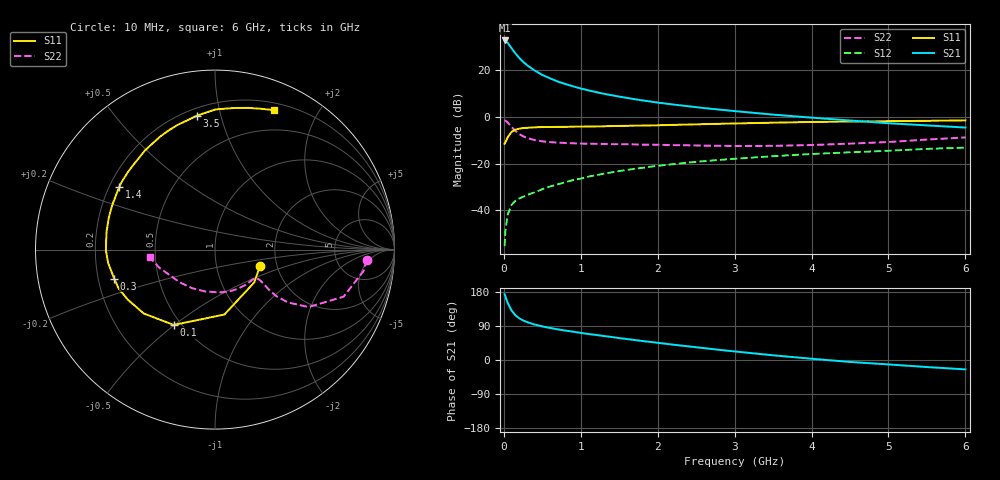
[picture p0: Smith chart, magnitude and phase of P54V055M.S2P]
! SIEMENS Small Signal Semiconductors
! BFP183
! Si NPN RF Bipolar Junction Transistor in SOT143
! VCE = 4 V  IC = 55 mA
! Common Emitter S-Parameters:  March  1996
# GHz  S  MA  R  50
!  f  S11  S21  S12  S22
! GHz  MAG  ANG  MAG  ANG  MAG  ANG  MAG  ANG
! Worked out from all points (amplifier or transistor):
!   36 points, 10 MHz to 6 GHz, reference 50 ohm
!   highest |S21| = 32.8 dB at 10 MHz (marker M1)
!   |S21| within 3 dB of that: start of sweep to 93.16 MHz
!   unconditionally stable (mu >= 1): start of sweep to 17.92 MHz; 311.2 MHz to end of sweep
!   at 250 MHz: K = 0.89, MSG = 28.9 dB, |S12| = -34.2 dB
!   at 1.4 GHz: K = 1.39, MAG = 12.8 dB, |S12| = -23.8 dB
!   at 6 GHz: K = 1.07, MAG = 2.7 dB, |S12| = -13.2 dB
!   S11 on the Smith chart (normalised r, x): 10 MHz: 1.63, -0.33; 100 MHz: 0.46, -0.50; 300 MHz: 0.27, -0.13; 1.4 GHz: 0.24, +0.28; 3.5 GHz: 0.25, +0.85; 6 GHz: 0.27, +1.47
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0.01  0.2669 -20.4  43.59 173.6  0.0017 72.9  0.8469 -3.8
0.02  0.285 -39.9  43.19 167.7  0.0036 72.5  0.8354 -8.3
0.05  0.3655 -81.7  38.92 150.5  0.0081 70.2  0.763 -20.1
0.1  0.4785 -118.7  29.74 130.7  0.013 54.0  0.6111 -31.6
0.15  0.5332 -138.1  23.05 118.2  0.016 51.0  0.5015 -35.9
0.2  0.5604 -150.2  18.42 110.1  0.0179 49.1  0.4302 -37.2
0.25  0.5786 -157.9  15.23 104.4  0.0194 51.7  0.385 -36.9
0.3  0.5844 -163.9  12.93 100.2  0.0211 53.2  0.3555 -36.0
0.4  0.5994 -172.6  9.901 93.6  0.0243 55.3  0.3198 -34.8
0.5  0.6075 -179.2  7.958 88.7  0.0283 56.2  0.3002 -34.2
0.6  0.6084 175.6  6.731 84.6  0.0323 58.8  0.2888 -34.2
0.7  0.6122 170.9  5.749 80.9  0.036 59.9  0.2812 -34.6
0.8  0.6138 167.1  5.073 77.6  0.0399 60.8  0.2766 -35.4
1.1  0.6241 156.2  3.714 68.6  0.0526 61.0  0.2664 -39.5
1.4  0.6375 146.9  2.925 60.8  0.0649 60.1  0.2618 -45.0
1.8  0.6532 135.4  2.267 50.1  0.0812 57.6  0.2551 -53.8
2.2  0.6762 125.3  1.848 40.5  0.0973 53.9  0.2492 -63.7
2.8  0.7124 111.2  1.439 26.8  0.1199 48.0  0.2412 -81.0
3.5  0.7531 97.6  1.122 12.4  0.1443 41.5  0.2399 -103.6
4.5  0.7958 82.4  0.838 -5.1  0.1747 31.5  0.2681 -137.1
5.5  0.8258 71.8  0.659 -18.6  0.2068 22.8  0.3279 -162.4
6  0.8437 67.1  0.593 -24.8  0.2198 17.8  0.3642 -173.2
